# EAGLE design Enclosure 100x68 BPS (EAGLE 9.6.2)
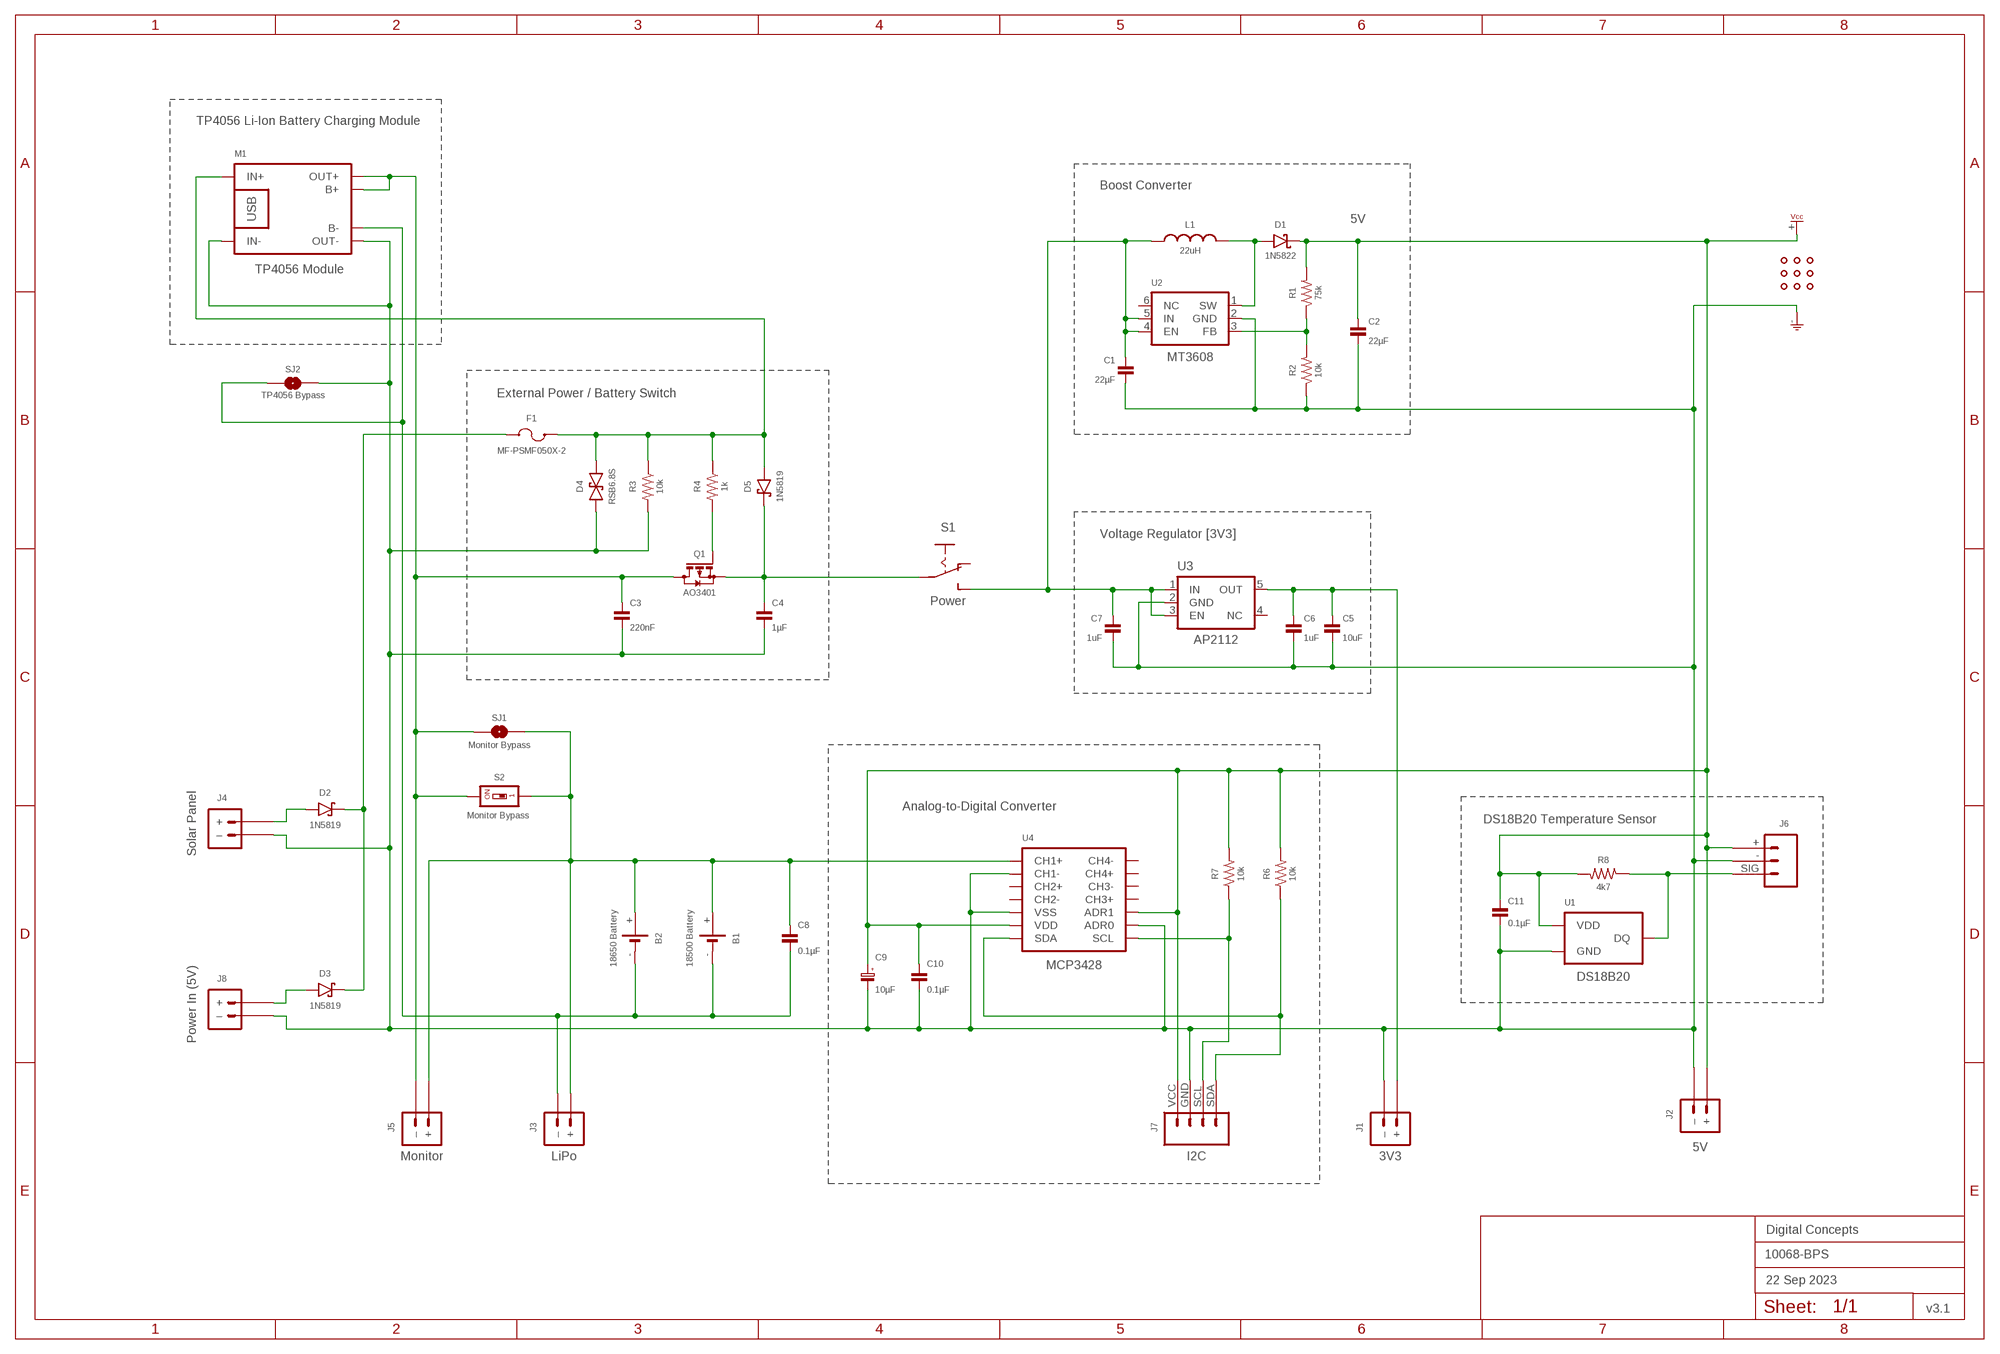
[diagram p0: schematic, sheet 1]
FRAME2 (A3L-LOC): DATE: 22 Sep 2023; OWNER: Digital Concepts; TITLE: 10068-BPS; VERSION: v3.1

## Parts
B1  18500 Battery  BATTERY-HOLDER-18500  [BATTERY-18500]
B2  18650 Battery  BATTERY-HOLDER-18650  [BATTERY-18650]
C1  22µF  CAPACITOR-1206  [C1206]
C2  22µF  CAPACITOR-1206  [C1206]
C3  220nF  CAPACITOR-0805  [C0805]
C4  1µF  CAPACITOR-0805  [C0805]
C5  10uF  CAPACITOR-0805  [C0805]
C6  1uF  CAPACITOR-0805  [C0805]
C7  1uF  CAPACITOR-0805  [C0805]
C8  0.1µF  CAPACITOR-0805  [C0805]
C9  10µF  CAPACITOR-1206-TANTALUM  [C1206-POLARISED]
C10  0.1µF  CAPACITOR-0805  [C0805]
C11  0.1µF  CAPACITOR-0805  [C0805]
D1  1N5822  DIODE-SCHOTTKY-1N5822  [DIODE_SMB]
D2  1N5819  DIODE-SCHOTTKY-1N5819  [SOD-123]
D3  1N5819  DIODE-SCHOTTKY-1N5819  [SOD-123]
D4  RSB6.8S  DIODE-BIDIRECTIONAL-RSB6.8S  [EMD2]
D5  1N5819  DIODE-SCHOTTKY-1N5819  [SOD-123]
F1  MF-PSMF050X-2  [F0805]
J1  3V3  JST-PH2.0-2-VERTICAL-POWER  [JST-PH2.0-2-VERTICAL-POWER]
J2  5V  JST-PH2.0-2-VERTICAL-POWER  [JST-PH2.0-2-VERTICAL-POWER]
J3  LiPo  JST-PH2.0-2-HORIZONTAL-POWERJST-PTH-2  [JST-PH2.0-2-HORIZONTAL-POWER]
J4  Solar Panel  JST-PH2.0-2-VERTICAL-POWER  [JST-PH2.0-2-VERTICAL-POWER]
J5  Monitor  JST-PH2.0-2-VERTICAL-POWER  [JST-PH2.0-2-VERTICAL-POWER]
J6  JST-PH2.0-3-HORIZONTAL-DS18B20  [JST-PH2.0-3-HORIZONTAL-DS18B20]
J7  I2C  JST-PH2.0-4-HORIZONTAL-I2C  [JST-PH2.0-4-HORIZONTAL-I2C]
J8  Power In (5V)  JST-GH1.25-2-HORIZONTAL-POWER  [JST-GH1.25-2-HORIZONTAL]
L1  22uH  INDUCTOR-CDRH104R+L5038P  [CDRH104R+]
M1  TP4056 Module  BATTERY-CHARGER-LI-PROT  [BATTERY-CHARGER-LI-PROT]
Q1  AO3401  MOSFET-AO3401  [SOT-23]
R1  75k  RESISTORR0805  [R0805]
R2  10k  RESISTORR0805  [R0805]
R3  10k  RESISTORR0805  [R0805]
R4  1k  RESISTORR0805  [R0805]
R6  10k  RESISTORR0805  [R0805]
R7  10k  RESISTORR0805  [R0805]
R8  4k7  RESISTORR0805  [R0805]
S1  Power  SWITCH-SLIDE-SPDT-PTH  [SWITCH-SPDT-PTH]
S2  Monitor Bypass  SWITCH-DIP-SWS001-VIA-1  [SMD-001-VIA-1]
SJ1  Monitor Bypass  SJ  [SJ]
SJ2  TP4056 Bypass  SJ  [SJ]
U1  DS18B20  THERMOMETER-DS18B20  [TO-92]
U2  MT3608  [SOT-23-6]
U3  AP2112  REGULATOR-AP2112  [SOT25]
U4  MCP3428  [SOIC-14]
U$1  PROTO-34X22-PI-CUT  [PROTO-34X22-PI-CUT]

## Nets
3V3: C5.1 C6.1 J1.+ U3.5(OUT)
5V: C2.1 C9.1(+) C10.1 C11.1 D1.C J2.+ J6.+ J7.VCC R1.2 R6.2 R7.2 R8.2 U1.3(VDD) U4.P$6(VDD) U4.P$10(ADR1) U$1.+(VCC)
GND: C1.2 C2.2 C3.2 C4.2 C5.2 C6.2 C7.2 C9.2(-) C10.2 C11.2 D4.P$2 J1.-(–) J2.-(–) J4.-(–) J6.- J7.GND J8.-(–) M1.IN- M1.OUT- R2.1 R3.2 SJ2.1 U1.1(GND) U2.2(GND) U3.2(GND) U4.P$2(CH1-) U4.P$5(VSS) U4.P$9(ADR0) U$1.-(GND)
N$1: D2.A J4.+
N$2: C1.1 C7.1 L1.2 S1.3(S) U2.4(EN) U2.5(IN) U3.1(IN) U3.3(EN)
N$4: R1.1 R2.2 U2.3(FB)
N$5: J7.SCL R7.1 U4.P$8(SCL)
N$6: D1.A L1.1 U2.1(SW)
N$7: D4.P$1 D5.A F1.2 M1.IN+ R3.1 R4.1
N$8: C4.1 D5.C Q1.2(S) S1.2(P)
N$10: B1.+ B2.+ C8.1 J3.+ J5.+ S2.1 S2.1@VIA SJ1.1 U4.P$1(CH1+)
N$11: D3.A J8.+
N$13: J6.SIG R8.1 U1.2(DQ)
N$15: J7.SDA R6.1 U4.P$7(SDA)
N$16: Q1.1(G) R4.2
N$17: C3.1 J5.-(–) M1.B+ M1.OUT+ Q1.3(D) S2.2 SJ1.2
N$38: B1.- B2.- C8.2 J3.-(–) M1.B- SJ2.2
N$41: D2.C D3.C F1.1
Unconnected: S1.1(O) U2.6(NC) U3.4(NC) U4.P$3(CH2+) U4.P$4(CH2-) U4.P$11(CH3+) U4.P$12(CH3-) U4.P$13(CH4+) U4.P$14(CH4-)

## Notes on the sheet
- TP4056 Li-Ion Battery Charging Module
- Boost Converter
- 5V
- External Power / Battery Switch
- Voltage Regulator [3V3]
- Analog-to-Digital Converter
- DS18B20 Temperature Sensor

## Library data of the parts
B1 = digitalconcepts:BATTERY-HOLDER-18500: 18500 Battery Holder
B2 = digitalconcepts:BATTERY-HOLDER-18650: 18650 Battery Holder
C1 C2 = digitalconcepts:CAPACITOR-1206: 1206 Capacitor
C3-C8 C10 C11 = digitalconcepts:CAPACITOR-0805: 0805 Capacitor
C9 = digitalconcepts:CAPACITOR-1206-TANTALUM: Capacitor 1206 Tantalum
D1 = digitalconcepts:DIODE-SCHOTTKY-1N5822: 1N5822 Schottky Diode SMB
D2 D3 D5 = digitalconcepts:DIODE-SCHOTTKY-1N5819: 1N5819 Schottky Diode SOD-123
D4 = digitalconcepts:DIODE-BIDIRECTIONAL-RSB6.8S: Schottky Bidirectional Diode
F1 = digitalconcepts:MF-PSMF050X-2: PTC Resettable Fuse
J1 J2 J4 J5 = digitalconcepts:JST-PH2.0-2-VERTICAL-POWER: JST PH2.0 2P PTH Connector (Power)
J3 = digitalconcepts:JST-PH2.0-2-HORIZONTAL-POWER: PH2.0 2P Right Angle PCB Connector; PROD_ID: CONN-09863; SKU: PRT-09914
J6 = digitalconcepts:JST-PH2.0-3-HORIZONTAL-DS18B20: DS18B20 PH2.0 Right Angle PCB Connector
J7 = digitalconcepts:JST-PH2.0-4-HORIZONTAL-I2C: PH2.0 4P Horizontal I2C
J8 = digitalconcepts:JST-GH1.25-2-HORIZONTAL-POWER: JST GH1.25 2P PTH Connector (Power)
L1 = digitalconcepts:INDUCTOR-CDRH104R+: Inductor; SPICEPREFIX: L
M1 = digitalconcepts:BATTERY-CHARGER-LI-PROT: TP4056 Li Battery Charger module with PCB (rather than module) footprint
Q1 = digitalconcepts:MOSFET-AO3401: AO3401 P-Channel MOSFET
R1-R4 R6-R8 = digitalconcepts:RESISTOR: Resistor; SPICEPREFIX: R
S1 = digitalconcepts:SWITCH-SLIDE-SPDT-PTH: Mini Sliding Switch SPDT PTH
S2 = digitalconcepts:SWITCH-DIP-SWS001-VIA-1: SMD Dip Switch 1 pol.
SJ1 SJ2 = digitalconcepts:SJ: Solder Jumper
U1 = digitalconcepts:THERMOMETER-DS18B20: Digital Thermometer -55C-125C TO92-3; AVAILABILITY: Bad; DESCRIPTION: Temperature Sensor Digital, Local -55°C ~ 125°C 12 b 8-uMAX; MF: Maxim Integrated; MP: DS18B20; PACKAGE: TO-92 Maxim Integrated; PRICE: None
U2 = digitalconcepts:MT3608: MT3608 DC-DC Step-Up Voltage Converter
U3 = digitalconcepts:REGULATOR-AP2112: Diodes Incorporated LDO Regulator with Enable; OC_FARNELL: unknown; OC_NEWARK: unknown
U4 = digitalconcepts:MCP3428: MCP3428 4 Channel ADC
U$1 = digitalconcepts:PROTO-34X22-PI-CUT: 34 x 22 Prototyping board, with Raspberyr Pi Zero mount points and power supply socket cut-out, to fit an 100 x 68 enclosure

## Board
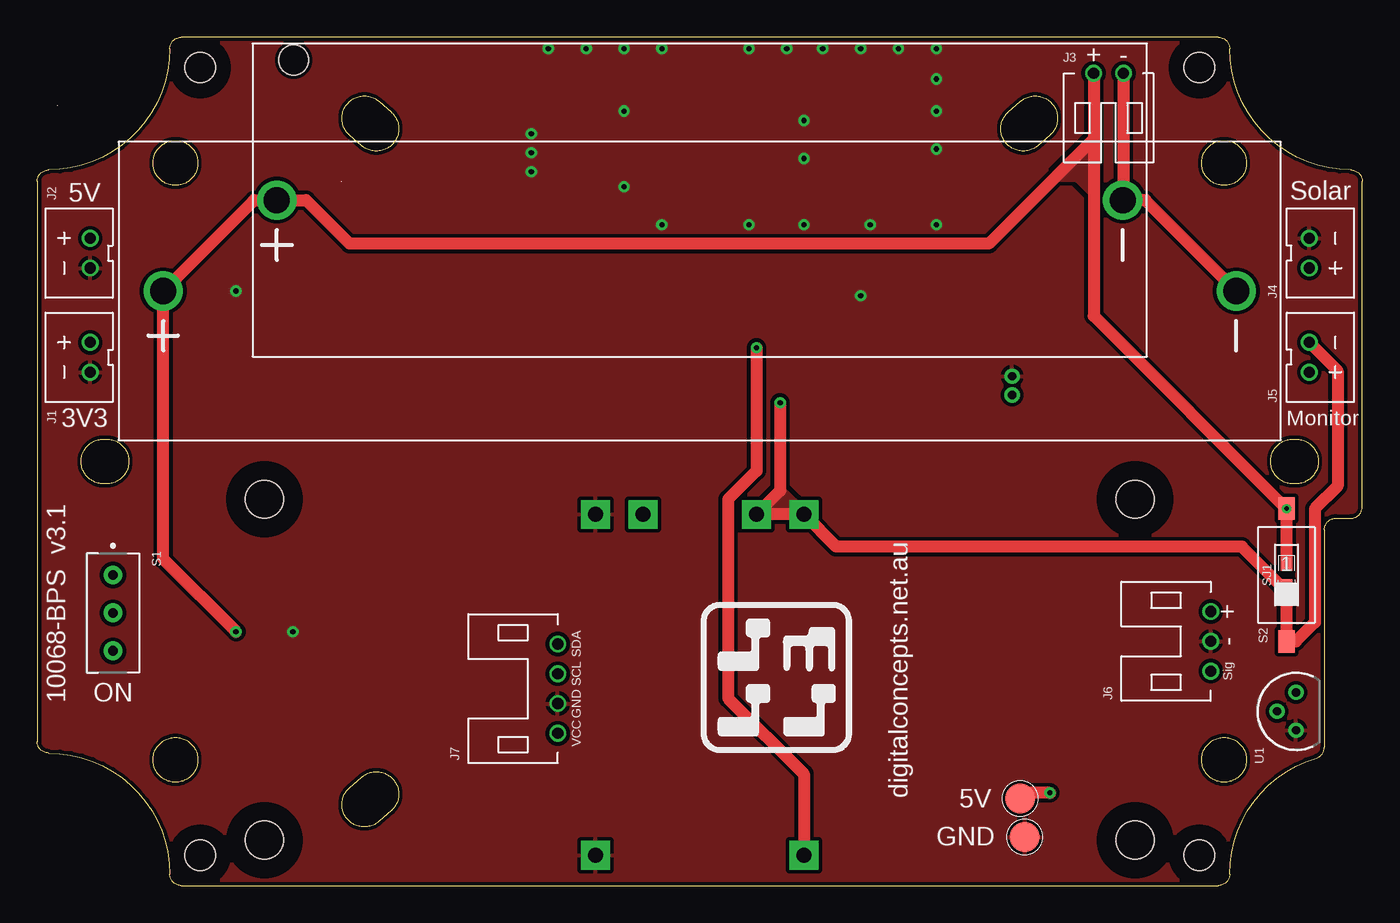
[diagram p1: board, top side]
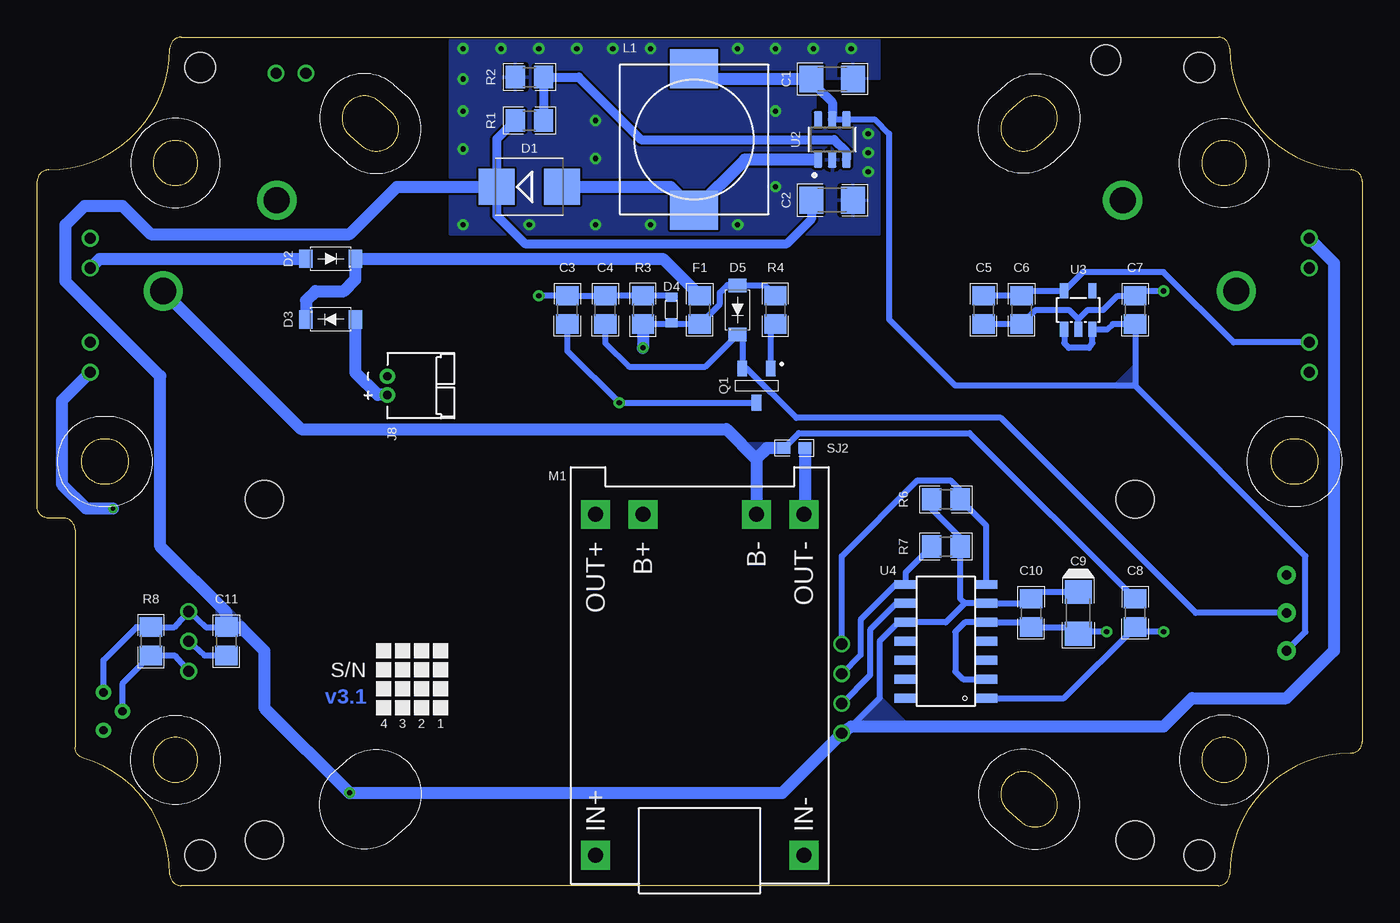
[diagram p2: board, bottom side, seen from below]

Size 88.9 x 56.9 mm. Coordinates in mm from the lower left corner, seen from the top.
Copper layers (1*16): Top 0.035mm / dielectric 1.5mm / Bottom 0.035mm
Design rules "default *": minimum track width 6mil, minimum drill 0.3mm, track to track 6mil, track to pad 6mil, pad to pad 6mil, via to via 6mil, smd to smd 6mil, copper to edge 6mil, drill to drill 6mil, minimum pad ring 1mil, minimum via ring 8mil, stop-mask expansion 4mil, vias tented up to drill 0mil, thermal gap 10mil

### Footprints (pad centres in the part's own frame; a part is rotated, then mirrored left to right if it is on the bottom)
BATTERY-18500 = drill 1.75: + -28.375,0; - 28.375,0 | hole 2: -27.25,9.4
BATTERY-18650 = drill 1.75: + -36,0; - 36,0
C1206 = smd 1.6 x 1.8: 1 -1.4,0; 2 1.4,0
C0805 = smd 1.3 x 1.5: 1 -0.95,0; 2 0.95,0
C1206-POLARISED = smd 1.6 x 1.8: 1 -1.4,0; 2 1.4,0
DIODE_SMB = smd 2.4 x 2.4: A 2.2,0; C -2.2,0
SOD-123 = smd 0.91 x 1.22: A -1.65,0; C 1.65,0
EMD2 = smd 0.6 x 0.8: P$1 -0.85,0; P$2 0.85,0
F0805 = smd 1.3 x 1.5: 1 -0.95,0; 2 0.95,0
JST-PH2.0-2-VERTICAL-POWER = drill 0.75: + -1,0; - 1,0
JST-PH2.0-2-HORIZONTAL-POWER = drill 0.75: + 1,0; - -1,0
JST-PH2.0-3-HORIZONTAL-DS18B20 = drill 0.75: + 2,0; - 0,0; SIG -2,0
JST-PH2.0-4-HORIZONTAL-I2C = drill 0.75: GND -1,0; SCL 1,0; SDA 3,0; VCC -3,0
JST-GH1.25-2-HORIZONTAL = drill 0.55 pad 1.016: + -0.625,0; - 0.625,0
CDRH104R+ = smd 2.6 x 3.2: 1 -4.75,0; 2 4.75,0
BATTERY-CHARGER-LI-PROT = drill 1 pad 1.93 square: B+ 10.795,3.81; B- 10.795,-3.81; IN+ -12.065,6.985; IN- -12.065,-6.985; OUT+ 10.795,6.985; OUT- 10.795,-6.985
SOT-23 = smd 0.65 x 1.05: 1 -0.95,-1.15; 2 0.95,-1.15; 3 0,1.15
R0805 = smd 1.3 x 1.5: 1 -0.95,0; 2 0.95,0
SWITCH-SPDT-PTH = drill 0.65 pad 1.27: 1 -2.54,0; 2 0,0; 3 2.54,0
SMD-001-VIA-1 = smd 1.1 x 1.5: 1 0,-4.45; 2 0,4.45 | drill 0.3 pad 0.61: 1@VIA 0,-4.45
SJ = smd 0.864 x 0.762: 1 -0.711,0; 2 0.711,0
TO-92 = drill 0.55 pad 1.016: 1 -1.27,0; 2 0,1.27; 3 1.27,0
SOT-23-6 = smd 1.1 x 0.6: 1 -1.35,0.95; 2 -1.35,0; 3 -1.35,-0.95; 4 1.35,-0.95; 5 1.35,0; 6 1.35,0.95
SOT25 = smd 0.55 x 1: 1 -0.95,-1.3; 2 0,-1.3; 3 0.95,-1.3; 4 0.95,1.3; 5 -0.95,1.3
SOIC-14 = smd 0.6 x 1.5: P$1 -3.815,-2.7; P$2 -2.54,-2.7; P$3 -1.27,-2.7; P$4 0,-2.7; P$5 1.27,-2.7; P$6 2.54,-2.7; P$7 3.81,-2.7; P$8 3.81,2.7; P$9 2.54,2.7; P$10 1.27,2.7; P$11 0,2.7; P$12 -1.27,2.7; P$13 -2.54,2.7; P$14 -3.81,2.7
PROTO-34X22-PI-CUT = smd 2 x 2: + 21.51,-22.6; - 21.81,-25.2 | hole 2.032: -33.528,26.416; 33.528,26.416; 33.528,-26.416; -33.528,-26.416 | hole 2.54: -29.21,-25.4; 29.21,-25.4; -29.21,-2.54; 29.21,-2.54

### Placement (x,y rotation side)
B1  44.45,45.97 0 top
B2  44.45,39.88 0 top
C1  35.56,54.1 0 bottom
C2  35.56,45.97 0 bottom
C3  53.34,38.61 90 bottom
C4  50.8,38.61 90 bottom
C5  25.4,38.61 270 bottom
C6  22.86,38.61 270 bottom
C7  15.24,38.61 90 bottom
C8  15.24,18.29 90 bottom
C9  19.05,18.29 270 bottom
C10  22.23,18.29 270 bottom
C11  76.2,16.38 270 bottom
D1  55.88,46.86 0 bottom
D2  69.22,42.04 0 bottom
D3  69.22,37.97 180 bottom
D4  46.36,38.61 90 bottom
D5  41.91,38.61 270 bottom
F1  44.45,38.61 270 bottom
J1  3.56,35.43 270 top
J2  3.56,42.42 270 top
J3  71.88,54.48 180 top
J4  85.34,42.42 90 top
J5  85.34,35.43 90 top
J6  78.74,16.38 90 top
J7  34.93,13.21 90 top
J8  65.41,33.53 90 bottom
L1  44.83,50.04 90 bottom
M1  44.45,14.1 90 bottom
Q1  40.64,33.53 180 bottom
R1  55.88,51.31 180 bottom
R2  55.88,54.23 0 bottom
R3  48.26,38.61 90 bottom
R4  39.37,38.61 270 bottom
R6  27.94,25.91 180 bottom
R7  27.94,22.73 0 bottom
R8  81.28,16.38 90 bottom
S1  5.08,18.29 270 top
S2  83.82,20.83 180 top
SJ1  83.82,20.83 270 top
SJ2  38.1,29.34 180 bottom
U1  84.45,11.68 90 top
U2  35.56,50.04 90 bottom
U3  19.05,38.61 0 bottom
U4  27.94,16.38 90 bottom
U$1  44.45,28.45 0 top

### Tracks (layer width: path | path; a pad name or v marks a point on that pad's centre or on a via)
3V3
  Bottom 0.406: C5.1 C6.1 22.51,39.91 U3.5 18.76,41.15 13.34,41.15 8.62,36.43 J1.+
5V  (via drill 0.35)
  Top 0.813: U$1.+ 66.34,6.22 v67.95,6.22
  Bottom 0.406: U1.3 84.45,15.11 82.23,17.33 R8.2 79.7,17.33 J6.+ 77.59,17.33 C11.1 | C9.1 21.78,19.69 C10.1 22.54,18.92 U4.P$6 26.67,18.92 | 26.67,18.92 27.94,17.65 U4.P$10 31.12,17.65 32.39,16.38 32.39,12.57 34.29,10.67 | R6.2 28.89,25.27 26.99,23.37 R7.2 26.99,19.24 26.67,18.92
  Bottom 0.61: C2.1 36.96,44.7 38.61,43.05 56.18,43.05 58.08,44.96 D1.C 58.08,50.06 R1.2
  Bottom 0.813: J2.+ 1.91,41.77 1.91,15.75 5.08,12.57 11.43,12.57 13.34,10.67 34.29,10.67 J7.VCC 38.91,6.22 v67.95,6.22 73.66,11.94 73.66,15.75 75.25,17.33 C11.1 76.2,18.29 80.64,22.73 80.64,34.16 87,40.51 87,44.32 85.73,45.59 83.19,45.59 81.28,43.69 67.95,43.69 64.77,46.86 D1.C
  pour Bottom (no thermals): 32.39,12.57 30.48,10.67 34.29,10.67
  pour Bottom (no thermals): 76.54,18.63 75.01,17.09 76.54,17.09
$X0
  cutout Bottom: 10.92,56.9 arc180 10.92,52.83 arc180
$X1
  cutout Bottom: 77.98,56.9 arc180 77.98,52.83 arc180
$X2
  cutout Bottom: 77.98,4.06 arc180 77.98,0 arc180
$X3
  cutout Bottom: 10.92,4.06 arc180 10.92,0 arc180
$X4
  cutout Top: 10.92,56.9 arc180 10.92,52.83 arc180
$X5
  cutout Top: 77.98,56.9 arc180 77.98,52.83 arc180
$X6
  cutout Top: 77.98,4.06 arc180 77.98,0 arc180
$X7
  cutout Top: 10.92,4.06 arc180 10.92,0 arc180
GND  (via drill 0.35)
  Bottom 0.406: D4.P$2 46.45,39.56 R3.2 C4.2 C3.2 v55.25,39.56 | C5.2 C6.2 21.91,38.61 19.69,38.61 19.05,37.97 | 19.05,37.97 18.42,38.61 17.38,38.61 16.43,39.56 C7.2 14.92,39.88 v13.34,39.88 | U3.2 19.05,37.97 | U4.P$2 26.79,13.84 27.3,14.36 27.3,17.02 26.67,17.65 U4.P$5 22.54,17.65 C10.2 19.5,17.34 19.12,16.95 | 19.12,16.95 C9.2 | U4.P$9 31.24,18.92 33.02,17.15 33.02,14.11 J7.GND | v17.15,17.02 19.05,17.02 19.12,16.95 | J6.- 77.7,15.43 C11.2
  Bottom 0.813: SJ2.1 37.39,24.97 M1.OUT-
  other vias: 33.15,50.42 33.15,49.15 33.15,47.88 39.37,51.94 47.75,44.32 39.37,56.13 51.44,48.77 41.91,56.13 50.29,56.13 39.37,46.86 41.91,44.32 47.75,56.13 52.7,56.13 55.25,56.13 57.79,56.13 36.83,56.13 34.29,56.13 60.33,56.13 51.44,51.31 60.33,54.1 60.33,49.4 60.33,51.94 51.44,44.32 60.33,44.32 55.88,44.32
  pour Top (isolate 0.254, rank 5): -2.97,59.46 -2.97,-2.6 91.81,-2.6 91.81,59.46
  pour Bottom (rank 2): 61.21,57.02 32.39,57.02 32.39,54.13 36.7,54.13 36.7,51.18 32.39,51.18 32.39,43.69 61.21,43.69
N$1
  Bottom 0.813: J4.+ 84.73,42.04 D2.A
N$2
  Bottom 0.406: U3.1 20,36.38 19.69,36.07 18.34,36.07 18.1,36.38 U3.3 17.11,37.3 16.75,37.66 C7.1 15.24,33.53 | U2.5 U2.4 32.7,51.39 31.75,50.43 31.75,37.97 27.3,33.53 15.24,33.53 | S1.3 3.81,17.02 3.81,22.1 15.24,33.53
  Bottom 0.61: C1.1 36.51,53.48 35.56,52.53 U2.5
  Bottom 0.813: L1.2 44.15,54.1 C1.1
  pour Bottom (no thermals): 15.24,33.53 15.24,34.8 16.51,33.53
N$4
  Bottom 0.61: U2.3 34.61,49.22 35.43,50.04 48.39,50.04 52.58,54.23 R2.2 R1.1
N$5
  Bottom 0.406: R7.1 30.64,20.98 U4.P$8 31.27,20.19 33.66,17.81 33.66,15.48 J7.SCL
N$6
  Bottom 0.152: U2.1 36.7,48.69
  Bottom 0.813: D1.A 46.41,46.86 L1.1 41.43,48.69 36.7,48.69
N$7  (via drill 0.35)
  Top 0.813: v48.26,36.07 48.26,27.81 46.36,25.91 46.36,12.57 51.44,7.49 M1.IN+
  Bottom 0.406: R3.1 46.45,37.66 D4.P$1 46.26,37.66 F1.2 43.1,39 43.1,39.77 42.6,40.27 D5.A 40.07,40.26 R4.1
  Bottom 0.813: R3.1 v48.26,36.07
N$8
  Bottom 0.406: C4.1 50.8,36.39 49.21,34.8 44.07,34.8 D5.C 41.59,36.64 Q1.2 41.28,34.68 37.97,31.37 24.26,31.37 11.18,18.29 S1.2
N$10  (via drill 0.35)
  Top 0.813: SJ1.1 S2.1@VIA 70.88,38.22 70.88,50.1 | J3.+ 70.88,50.1 | 70.88,50.1 63.84,43.05 20.96,43.05 18.03,45.97 B1.+ 14.55,45.97 B2.+ 8.45,21.9 v13.34,17.02
  Bottom 0.406: U4.P$1 20.01,12.57 C8.1 14.92,17.02 v13.34,17.02
  Bottom 0.813: S2.1@VIA 85.6,25.28 87.25,26.93 87.25,32.53 J5.+
  pour Top (no thermals): 70.88,46.51 69.83,47.56 68.34,47.56 70.88,50.1
N$11
  Bottom 0.813: D3.A 67.56,34.43 66.04,32.9 J8.+
N$13
  Bottom 0.406: U1.2 83.19,13.53 R8.1 79.7,15.43 J6.SIG
N$15
  Bottom 0.406: U4.P$7 25.24,24.16 R6.1 26.99,26.54 27.62,27.18 29.84,27.18 34.93,22.1 J7.SDA
N$16
  Bottom 0.406: R4.2 39.69,37.34 Q1.1
N$17  (via drill 0.35)
  Top 0.813: J5.- 87.25,34.53 87.25,26.8 85.73,25.27 85.73,17.65 84.45,16.38 S2.2 SJ1.2 83.44,20.12 80.82,22.73 53.59,22.73 M1.OUT+ M1.B+ 49.85,26.48 v49.85,32.38
  Bottom 0.406: Q1.3 v49.85,32.38 53.34,35.87 C3.1
  pour Top (no thermals): 48.26,24.89 49.85,26.48 51.44,24.89
N$38
  Top 0.813: B2.- 74.35,45.97 B1.- 72.88,46.03 J3.-
  Bottom 0.406: SJ2.2 37.8,30.35 26.36,30.35 C8.2
  Bottom 0.813: B2.- 71.18,30.61 42.67,30.61 40.64,28.58 | SJ2.2 39.95,29.34 40.64,28.65 40.64,28.58 | 40.64,28.58 M1.B-
  pour Bottom: 39.95,29.34 41.33,29.34 40.64,28.7
N$41
  Bottom 0.813: D3.C 70.86,39.24 70.23,39.88 68.33,39.88 67.56,40.64 D2.C 46.93,42.04 F1.1

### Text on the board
Bottom: v3.1
tPlace: 10068-BPS v3.1 | digitalconcepts.net.au
bPlace: S/N | 1 | 2 | 3 | 4
tNames: Solar | ON | 5V | GND
tValues: Monitor Bypass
